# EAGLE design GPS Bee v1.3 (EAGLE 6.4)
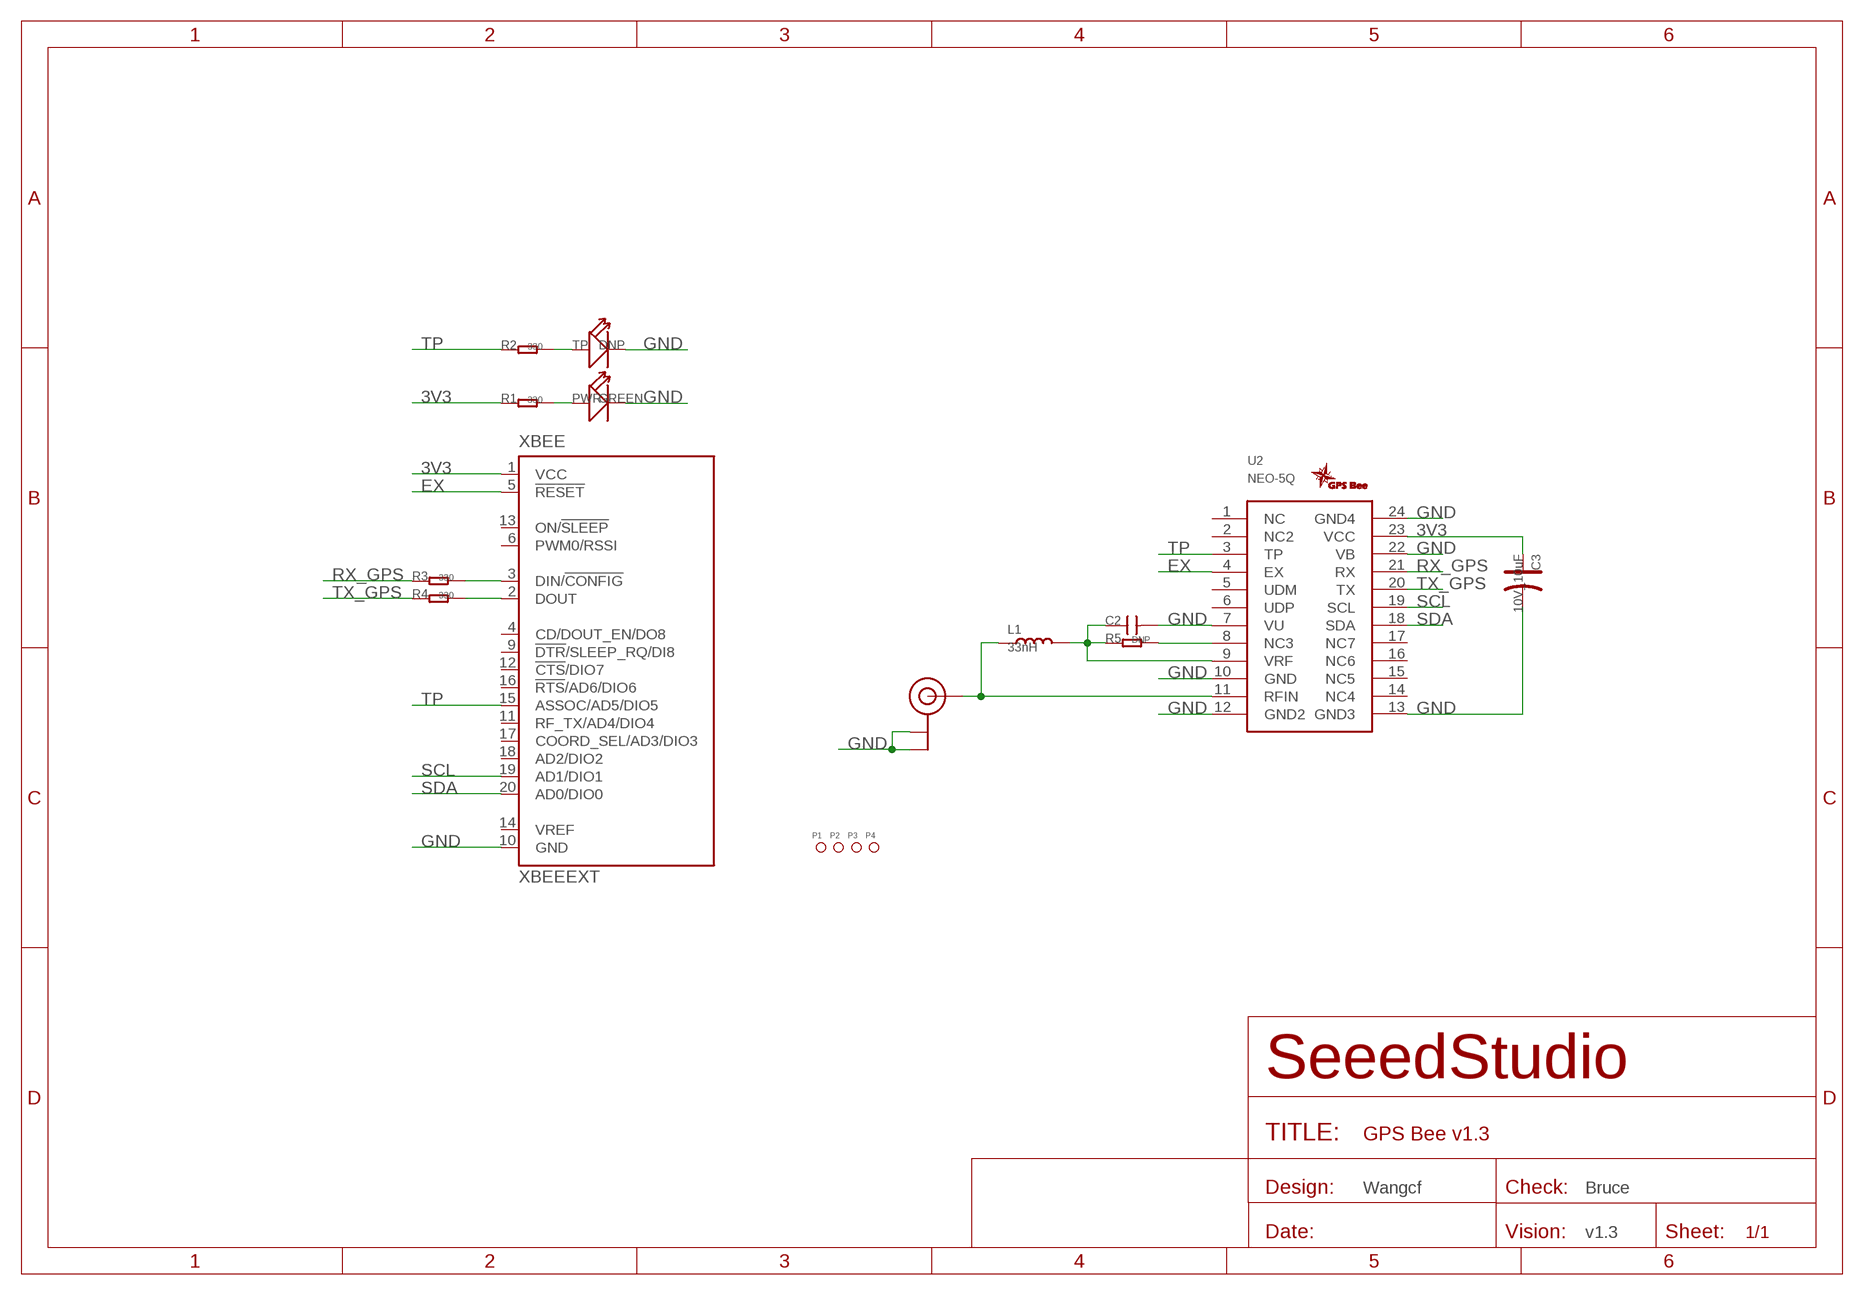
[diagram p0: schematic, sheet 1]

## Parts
C2  C-0603  [0603]
C3  10V_10uF  CAP-AVX-A  [AVX-A]
L1  33nH  L0603  [0603]
LOGO1  GPSLOGO_SLIK  [GPSLOGO]
P1  PAD-MARK  [ROUND-MARK-1.0]
P2  PAD-MARK  [ROUND-MARK-1.0]
P3  PAD-MARK  [ROUND-MARK-1.0]
P4  PAD-MARK  [ROUND-MARK-1.0]
PWR  GREEN  LED'RIGHT'  [LED-SIDE-VIEW-0603-RIGHT]
R1  330  R-0603  [0603]
R2  330  R-0603  [0603]
R3  330  R-0603  [0603]
R4  330  R-0603  [0603]
R5  DNP  R-0603  [0603]
TP  DNP  LED'RIGHT'  [LED-SIDE-VIEW-0603-RIGHT]
U2  NEO-5Q  [NEO-5Q]
U3  U.FL  [U.FL]
XBEE  XBEEEXT  [XBEE_PLUG]

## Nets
3V3: C3.+ R1.1 U2.23(VCC) XBEE.1(VCC)
EX: U2.4(EX) XBEE.5(!RESET)
GND: C2.2 C3.- PWR.2(-) TP.2(-) U2.7(VU) U2.10(GND) U2.12(GND2) U2.13(GND3) U2.22(VB) U2.24(GND4) U3.P$1(GND) U3.P$2(GND) XBEE.10(GND)
N$1: PWR.1(+) R1.2
N$2: L1.1 U2.11(RFIN) U3.P$3(SIGNAL)
N$3: C2.1 L1.2 R5.1 U2.9(VRF)
N$4: R3.2 XBEE.3(DIN/!CONFIG)
N$5: R2.2 TP.1(+)
N$6: R4.2 XBEE.2(DOUT)
N$7: R5.2 U2.8(NC3)
RX_GPS: R3.1 U2.21(RX)
SCL: U2.19(SCL) XBEE.19(AD1/DIO1)
SDA: U2.18(SDA) XBEE.20(AD0/DIO0)
TP: R2.1 U2.3(TP) XBEE.15(ASSOC/AD5/DIO5)
TX_GPS: R4.1 U2.20(TX)
Unconnected: U2.1(NC) U2.2(NC2) U2.5(UDM) U2.6(UDP) U2.14(NC4) U2.15(NC5) U2.16(NC6) U2.17(NC7) XBEE.4(CD/DOUT_EN/DO8) XBEE.6(PWM0/RSSI) XBEE.9(!DTR!/SLEEP_RQ/DI8) XBEE.11(RF_TX/AD4/DIO4) XBEE.12(!CTS!/DIO7) XBEE.13(ON/!SLEEP) XBEE.14(VREF) XBEE.16(!RTS!/AD6/DIO6) XBEE.17(COORD_SEL/AD3/DIO3) XBEE.18(AD2/DIO2)

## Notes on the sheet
- Wangcf | Bruce
- v1.3

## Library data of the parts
C2 = Discrete:C*: Ceramic Capacitors
C3 = Discrete:CAP*: Electrolytic Capacitors,Tantalum Capacitors and Super Capacitors
L1 = Discrete:L*
LOGO1 = logo:GPSLOGO_SLIK
P1-P4 = Discrete:PAD-MARK; PARTNO: DNP
PWR TP = Discrete:LED*
R1-R5 = Discrete:R*
U2 = Seeed:NEO-5Q
U3 = SparkFun2:U.FL
XBEE = EXT_moudle:XBEE: XBee (TM) /XBee-PRO(TM) OEM RF Modules Source: MaxStream, Inc. xbee_productmanual.pdf

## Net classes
0 default: width 0.003 mm, drill 0.254 mm, clearance 0.152 mm

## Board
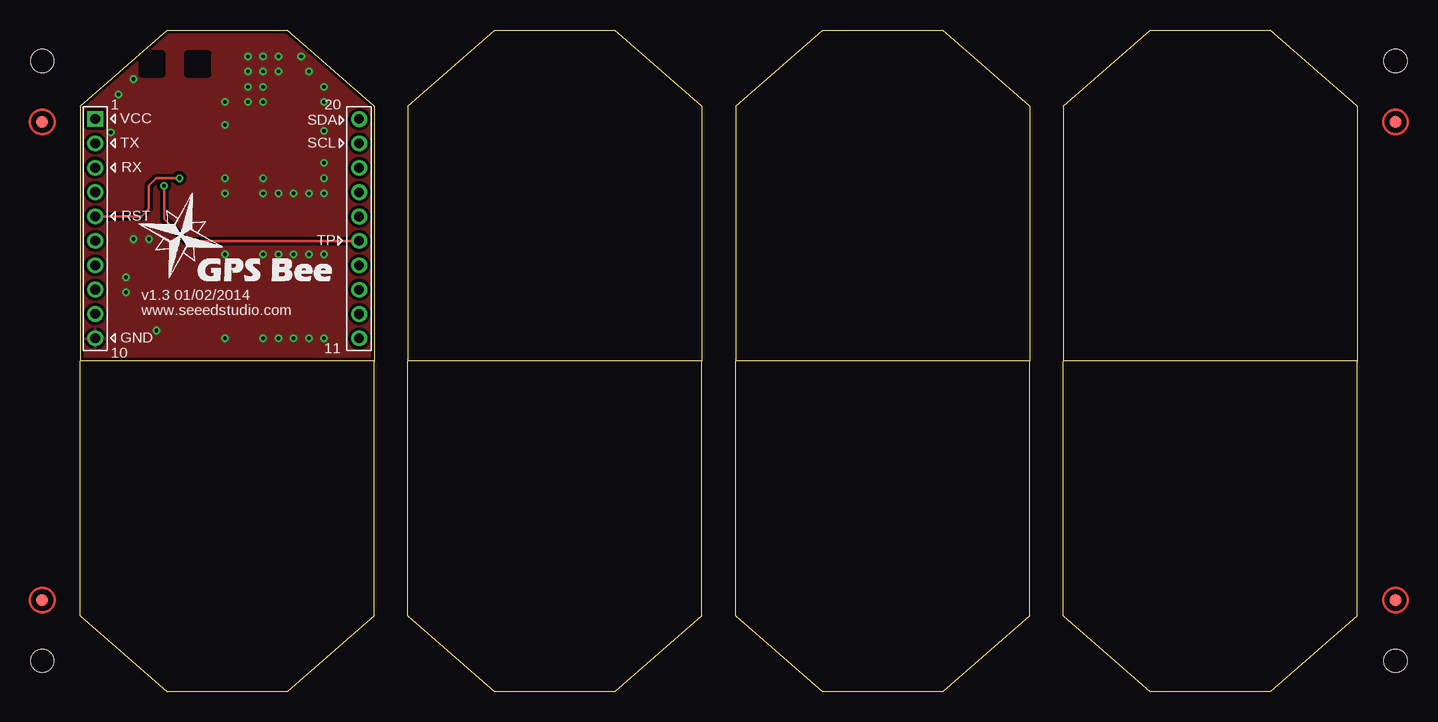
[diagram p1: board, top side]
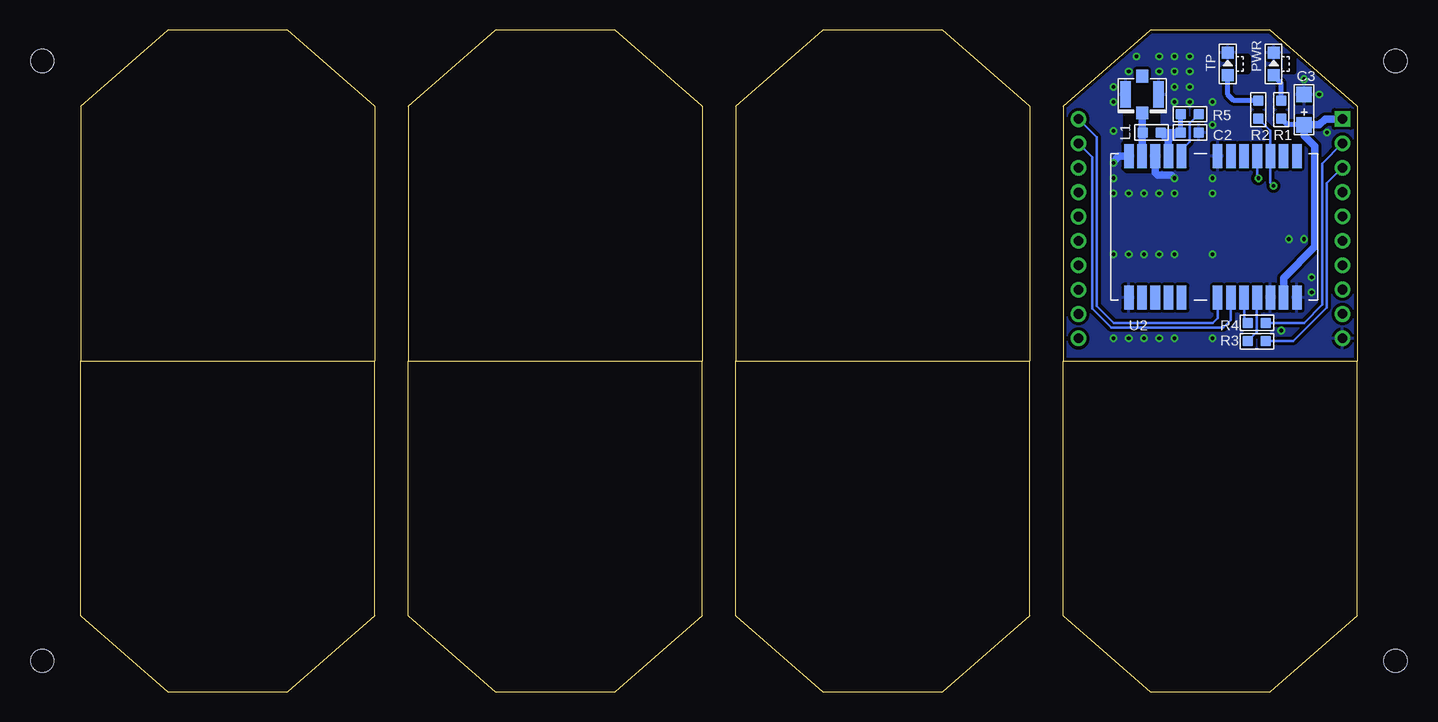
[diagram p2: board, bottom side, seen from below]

Size 106.41 x 55.2 mm. Coordinates in mm from the lower left corner, seen from the top.
Outline: 0,27.6 0,48.85 7.25,55.2 17.25,55.2 24.5,48.85 24.5,27.6
Outline: 27.31,27.6 27.31,48.85 34.56,55.2 44.56,55.2 51.81,48.85 51.81,27.6
Outline: 54.61,27.6 54.61,48.85 61.86,55.2 71.86,55.2 79.11,48.85 79.11,27.6
Outline: 81.92,27.6 81.92,48.85 89.17,55.2 99.17,55.2 106.42,48.85 106.42,27.6
Outline: 24.5,27.6 24.5,6.35 17.25,0 7.25,0 0,6.35 0,27.6
Outline: 24.5,27.6 0,27.6
Outline: 51.81,27.6 51.81,6.35 44.56,0 34.56,0 27.31,6.35 27.31,27.6
Outline: 51.81,27.6 27.31,27.6
Outline: 79.11,27.6 79.11,6.35 71.86,0 61.86,0 54.61,6.35 54.61,27.6
Outline: 79.11,27.6 54.61,27.6
Outline: 106.42,27.6 106.42,6.35 99.17,0 89.17,0 81.92,6.35 81.92,27.6
Outline: 106.42,27.6 81.92,27.6
Copper layers (1*16): Top 0.035mm / dielectric 1.5mm / Bottom 0.035mm
Design rules "default": minimum track width 6mil, minimum drill 12mil, track to track 6mil, track to pad 6mil, pad to pad 6mil, via to via 6mil, smd to smd 0mil, copper to edge 10mil, drill to drill 10mil, minimum pad ring 10mil, minimum via ring 6mil, stop-mask expansion 2mil, vias tented up to drill 100mil, thermal gap 10mil
Holes 1.91 mm at -3.17,2.58 -3.17,52.62 109.61,52.62 109.61,2.58
tRestrict: area 8.9,51.5 to 10.7,53.3; area 5.1,51.5 to 6.9,53.3
bRestrict: area 5.3,51.7 to 6.6,53; area 9.2,51.7 to 10.4,53; 4 lines

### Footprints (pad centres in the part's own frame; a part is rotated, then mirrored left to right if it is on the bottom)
0603 = smd 0.889 x 0.889: 1 -0.762,0; 2 0.762,0
AVX-A = smd 1.27 x 1.27: + -1.27,0; - 1.27,0
ROUND-MARK-1.0 = smd 1.016 x 1.016: P$1 0,0
LED-SIDE-VIEW-0603-RIGHT = smd 1 x 1: 1 0,-0.95; 2 0,0.95
NEO-5Q = smd 2 x 0.8: 1 12,-14; 2 12,-12.9; 3 12,-11.8; 4 12,-10.7; 5 12,-9.6; 6 12,-8.5; 7 12,-7.4; 8 12,-4.4; 9 12,-3.3; 10 12,-2.2; 11 12,-1.1; 12 12,0; 13 0.2,0; 14 0.2,-1.1; 15 0.2,-2.2; 16 0.2,-3.3; 17 0.2,-4.4; 18 0.2,-7.4; 19 0.2,-8.5; 20 0.2,-9.6; 21 0.2,-10.7; 22 0.2,-11.8; 23 0.2,-12.9; 24 0.2,-14
U.FL = smd 2.2 x 0.85: P$1 0,1.375; P$2 0,-1.375 | smd 1.05 x 1: P$3 1.525,0; P$4 -1.525,0
XBEE_PLUG = drill 0.8 pad 1.27 square: 1 0,0.008 | drill 0.8 pad 1.27: 2 0,-2.024; 3 0,-4.056; 4 0,-6.088; 5 0,-8.12; 6 0,-10.152; 7 0,-12.184; 8 0,-14.216; 9 0,-16.248; 10 0,-18.28; 11 21.996,-18.288; 12 21.996,-16.256; 13 21.996,-14.224; 14 21.996,-12.192; 15 21.996,-10.16; 16 21.996,-8.128; 17 21.996,-6.096; 18 21.996,-4.064; 19 21.996,-2.032; 20 21.996,0

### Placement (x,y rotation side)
C2  13.98,46.65 0 bottom
C3  4.45,48.55 90 bottom
L1  17.15,46.65 0 bottom
LOGO1  4.45,33.31 0 top
P1  not placed on the board
P2  not placed on the board
P3  not placed on the board
P4  not placed on the board
PWR  6.99,52.37 0 bottom
R1  6.36,48.55 90 bottom
R2  8.26,48.55 90 bottom
R3  8.39,29.25 0 bottom
R4  8.39,30.78 0 bottom
R5  13.98,48.17 0 bottom
TP  10.8,52.37 0 bottom
U2  19.06,32.68 90 bottom
U3  17.96,49.83 270 bottom
XBEE  1.25,47.77 0 top

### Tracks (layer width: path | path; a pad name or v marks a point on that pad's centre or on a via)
3V3
  Bottom 0.406: C3.+ 5.85,47.28 R1.1
  Bottom 0.61: XBEE.1 2.69,47.78 3.18,47.28 C3.+ 4.45,46.4 3.56,45.51 3.56,37.12 6.16,34.53 U2.23
EX  (via drill 0.3 pad 0.64)
  Top 0.203: XBEE.5 5.07,39.65 5.72,40.3 5.72,42.2 6.36,42.84 v8.26,42.84
  Bottom 0.203: U2.4 8.36,42.94 v8.26,42.84
GND  (via drill 0.3 pad 0.64)
  Bottom 0.61: U2.12 19.88,44.68 20.33,44.24 v20.33,44.11 | U2.10 16.86,43.31 16.64,43.09 15.5,43.09 v15.25,42.84
  other vias: 15.25,49.19 15.25,50.46 15.25,51.73 16.52,51.73 20.33,50.46 20.33,49.19 20.33,42.84 19.06,41.57 17.79,41.57 16.52,41.57 15.25,41.57 20.33,46.78 19.06,51.73 20.33,41.57 3.82,34.59 5.72,37.76 3.82,33.31 4.45,37.76 19.06,36.49 12.07,42.84 12.07,41.57 12.07,47.28 12.07,49.19 15.25,36.49 3.18,49.83 4.45,51.09 13.98,49.19 13.98,50.46 13.98,51.73 18.42,53 16.52,53 15.25,53 13.98,53 17.79,36.49 20.33,36.49 16.52,36.49 12.07,36.49 6.36,30.14 12.07,29.51 15.25,29.51 16.52,29.51 17.79,29.51 19.06,29.51 20.33,29.51 2.55,46.65
  pour Bottom (isolate 0.254): 0.01,55.54 24.77,55.54 24.77,27.6 0.01,27.6
  pour Top (isolate 0.254): 0.01,55.54 24.77,55.54 24.77,27.6 0.01,27.6
N$1
  Bottom 0.406: R1.2 6.36,50.78 PWR.1
N$2
  Bottom 0.61: U3.P$3 U2.11 17.96,46.61 L1.1
N$3
  Bottom 0.406: C2.1 R5.1
  Bottom 0.61: U2.9 15.76,46.02 | 15.76,46.02 L1.2 15.12,46.65 | C2.1 14.87,46.65 15.12,46.65 | 15.12,46.65 15.76,46.02
N$4
  Bottom 0.203: XBEE.3 2.55,42.42 2.55,32.05 5.34,29.25 R3.2
N$5
  Bottom 0.406: R2.2 10.29,49.32 10.8,49.83 TP.1
N$6
  Bottom 0.203: R4.2 4.45,30.78 2.93,32.3 2.93,44.07 XBEE.2
N$7
  Bottom 0.203: U2.8 14.66,45.21 13.98,45.89 13.98,47.41 R5.2
RX_GPS
  Bottom 0.203: U2.21 8.36,32.08 8.39,32.05 8.39,30.01 R3.1
SCL
  Bottom 0.203: U2.19 10.56,31.02 11.18,30.39 20.53,30.39 22.11,31.97 22.11,44.59 XBEE.19
SDA
  Bottom 0.203: U2.18 11.66,31.19 12.07,30.78 20.33,30.78 21.72,32.17 21.72,46.24 XBEE.20
TP  (via drill 0.3 pad 0.64)
  Top 0.203: XBEE.15 8.8,37.61 6.99,39.41 v6.99,42.2
  Bottom 0.203: R2.1 7.26,46.79 U2.3 7.26,42.47 v6.99,42.2
TX_GPS
  Bottom 0.203: U2.20 9.46,31.08 R4.1

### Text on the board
tPlace: 1 | 20 | VCC | SDA | TX | SCL | RX | RST | TP | v1.3 01/02/2014 | www.seeedstudio.com | GND | 11 | 10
